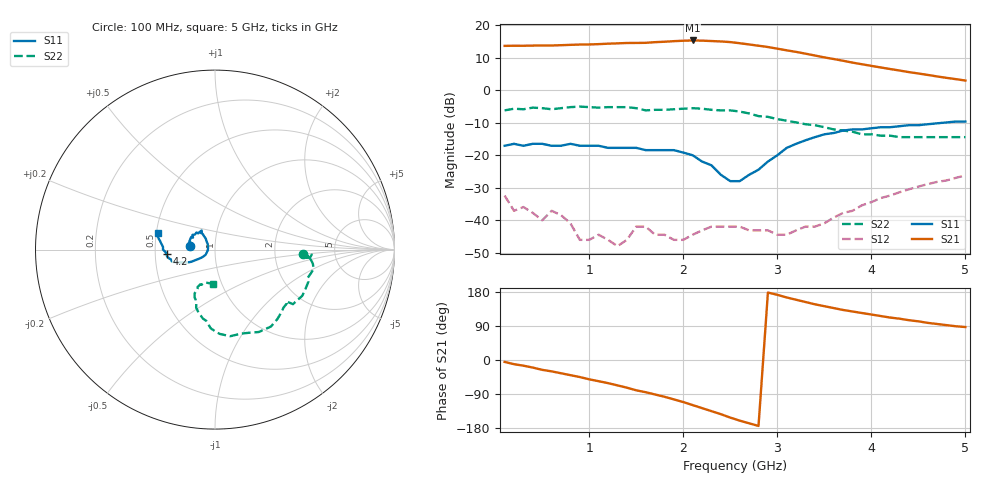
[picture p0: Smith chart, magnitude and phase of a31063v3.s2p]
!  INA-31063  S PARAMETERS
!  Vd = 3 V  LAST UPDATED 04-16-98
# ghz s ma r 50
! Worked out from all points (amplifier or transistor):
!   50 points, 100 MHz to 5 GHz, reference 50 ohm
!   highest |S21| = 15.3 dB at 2.1 GHz (marker M1)
!   |S21| within 3 dB of that: start of sweep to 3.093 GHz
!   unconditionally stable (mu >= 1): start of sweep to end of sweep
!   at 900 MHz: K = 13.43, MAG = 15.7 dB, |S12| = -46.0 dB
!   at 2.6 GHz: K = 9.23, MAG = 15.6 dB, |S12| = -41.9 dB
!   at 5 GHz: K = 6.31, MAG = 3.6 dB, |S12| = -26.2 dB
!   S11 on the Smith chart (normalised r, x): 100 MHz: 0.76, +0.03; 4.2 GHz: 0.58, -0.03; 5 GHz: 0.51, +0.10
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0.1  0.14 171.0  4.81 -5.0  0.024 10.0  0.49 -3.0
0.2  0.15 167.0  4.84 -11.0  0.014 11.0  0.52 -4.0
0.5  0.15 152.0  4.88 -26.0  0.01 -6.0  0.53 -5.0
0.6  0.14 152.0  4.88 -30.0  0.014 -18.0  0.51 -5.0
0.9  0.14 143.0  5.04 -45.0  0.005 -35.0  0.56 -11.0
1  0.14 138.0  5.06 -51.0  0.005 -4.0  0.55 -14.0
1.2  0.13 136.0  5.2 -61.0  0.005 -16.0  0.55 -19.0
1.4  0.13 129.0  5.33 -73.0  0.005 40.0  0.55 -28.0
1.5  0.13 125.0  5.34 -80.0  0.008 58.0  0.53 -35.0
1.8  0.12 130.0  5.57 -97.0  0.006 31.0  0.5 -40.0
2  0.11 128.0  5.77 -111.0  0.005 61.0  0.52 -48.0
2.1  0.1 129.0  5.83 -119.0  0.006 74.0  0.53 -54.0
2.4  0.05 144.0  5.63 -143.0  0.008 76.0  0.49 -73.0
2.5  0.04 166.0  5.5 -152.0  0.008 74.0  0.49 -80.0
2.6  0.04 -176.0  5.29 -160.0  0.008 76.0  0.47 -87.0
2.9  0.08 -149.0  4.62 178.0  0.007 86.0  0.39 -100.0
3.1  0.13 -152.0  4.11 165.0  0.006 105.0  0.34 -108.0
3.4  0.19 -158.0  3.42 147.0  0.008 125.0  0.29 -113.0
3.7  0.24 -163.0  2.84 132.0  0.013 144.0  0.24 -114.0
4.2  0.27 -175.0  2.12 112.0  0.024 154.0  0.2 -108.0
4.6  0.3 174.0  1.72 98.0  0.036 152.0  0.19 -99.0
5  0.33 164.0  1.41 87.0  0.049 150.0  0.19 -93.0
